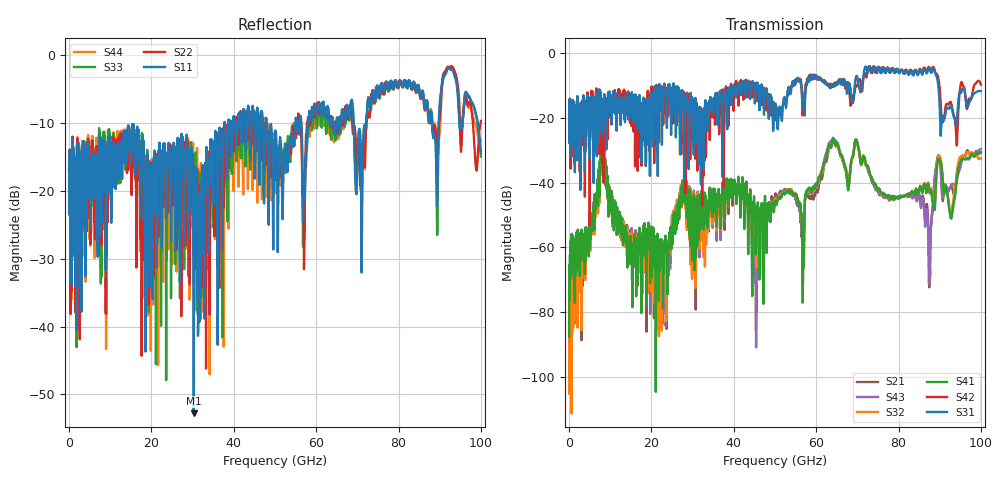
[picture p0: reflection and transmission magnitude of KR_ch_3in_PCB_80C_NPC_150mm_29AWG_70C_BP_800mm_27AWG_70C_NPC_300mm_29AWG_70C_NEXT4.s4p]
# GHz S RI R 45
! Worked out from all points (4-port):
!   4000 points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, 25 MHz to 100 GHz, reference 45 ohm
!   strongest paths, dB at 25 MHz, 25.02 GHz, 50.02 GHz, 75.03 GHz, 100 GHz:
!     S31: -20.6, -14.0, -16.2, -5.1, -11.8
!     S42: -20.7, -17.7, -18.0, -4.4, -9.7
!     S41: -87.6, -55.9, -45.5, -41.9, -30.7
!     S32: -105.1, -50.7, -44.9, -42.0, -32.5
!     S43: -101.4, -52.0, -44.8, -42.6, -29.6
!     S21: -102.2, -53.3, -44.8, -42.7, -30.6
!   lowest |S11| = -52.8 dB at 30.3 GHz (marker M1), VSWR 1.00, Z = 44.8 - j0.0223 ohm
!   |S11| at or under -10 dB: start of sweep to 37.74 GHz; 48.04 GHz to 54.97 GHz (6.937 GHz wide, 13.5 % of centre); 69.08 GHz to 72.18 GHz (3.105 GHz wide, 4.4 % of centre)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
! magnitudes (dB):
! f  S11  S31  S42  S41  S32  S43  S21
! 25 MHz  -16.6  -20.6  -20.7  -87.6  -105.1  -101.4  -102.2
! 8.1 GHz  -17.5  -25.5  -22.8  -25.2  -25.6  -25.1  -25.7
! 23 GHz  -13.7  -11.7  -15.3  -67.6  -63.8  -72.1  -72.1
! 30.3 GHz  -52.8  -31.4  -19.7  -45.0  -43.7  -43.4  -43.7
! 64.28 GHz  -10.2  -10.4  -9.8  -26.9  -27.6  -26.4  -27.6
! 87.55 GHz  -9.9  -4.8  -4.7  -43.2  -42.9  -63.4  -60.9
! 100 GHz  -14.3  -11.8  -9.7  -30.7  -32.5  -29.6  -30.6
